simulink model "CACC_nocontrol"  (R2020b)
settings: Solver=FixedStepAuto  StartTime=0.0  StopTime=runtime  FixedStep=stepsize  RelTol=1e-3
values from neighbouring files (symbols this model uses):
  A = [[A_l zeros(3)];[zeros(3) A_f]]    [set_CACC_nocontrol.m]
  A_22s = -eye(4)*0.1    [set_CACC_nocontrol.m]
  A_c = -1/h    (= -1.42857142857)    [set_CACC_nocontrol.m]
  attack_dur = 10    [set_CACC_nocontrol.m]
  attack_mag = 2.8    [set_CACC_nocontrol.m]    (also in Simulation_Main.m = sweep)
  attack_time = 2    [set_CACC_nocontrol.m]
  B = [[B_l zeros(3,1)];[zeros(3,1) B_f]]    [set_CACC_nocontrol.m]
  B_c = [kp/h kd/h -kp -kd]    [set_CACC_nocontrol.m]
  C = [[1 0 0 -1 0 0];[0 1 0 0 -1 0];[0 0 0 0 1 0];[0 0 0 0 0 1]]    [set_CACC_nocontrol.m]
  C_c = 1    [set_CACC_nocontrol.m]
  const = kp/h*r    (= 0.428571428571)    [set_CACC_nocontrol.m]
  D_c = [1/h 0]    [set_CACC_nocontrol.m]
  e2dot_max = diag(M)+U_max    [set_CACC_nocontrol.m]
  e2dot_min = diag(M)-U_max    [set_CACC_nocontrol.m]
  input_mag = 1    [set_CACC_nocontrol.m]
  input_time = [1 6]    [set_CACC_nocontrol.m]
  K = 0.1*eye(4)    [set_CACC_nocontrol.m]    (also in Simulation_Main.m = parameters{1}{2})
  L_f = 4    [set_CACC_nocontrol.m]
  M = diag([2.3500 3.300 2.160 3.6000])    [set_CACC_nocontrol.m]    (also in Simulation_Main.m = parameters{1}{1})
  r = 1.5    [set_CACC_nocontrol.m]
  r_e = e2dot_max./e2dot_min    [set_CACC_nocontrol.m]
  stepsize = 1/1000    (= 0.001)    [set_CACC_nocontrol.m]
  t_max = 2*F*zeta2_max./e2dot_min    [set_CACC_nocontrol.m]
  Thatx_0 = [zeros(2,1);temp(3:end)]    [set_CACC_nocontrol.m]
  U_max = abs(A_22s*obs.F)*abs(zeta2_max)+     abs((obs.A_22-A_22s)*obs.F)*abs(zeta2_max)+     abs(obs.E_2)*abs(zeta1_max)+     abs(obs.A_21*pinv(obs.A_11)*obs.A_12*obs.F)*abs(zeta2_max)+     abs(obs.A_21*pinv(obs.A_11)*obs.E_1)*abs(zeta1_max)    [set_CACC_nocontrol.m]
  x_0 = [-40;15;0;-50;15;0]    [set_CACC_nocontrol.m]
  zeta1_max = abs(tau_l/obs.hattau_l-1)*2*maxacc_l    [set_CACC_nocontrol.m]
  zeta2_max = 3*sqrt(sensor.var)    [set_CACC_nocontrol.m]
undefined symbols (not defined in the file or in its folder): obs, pinv, sensor
libraries: simulink x3

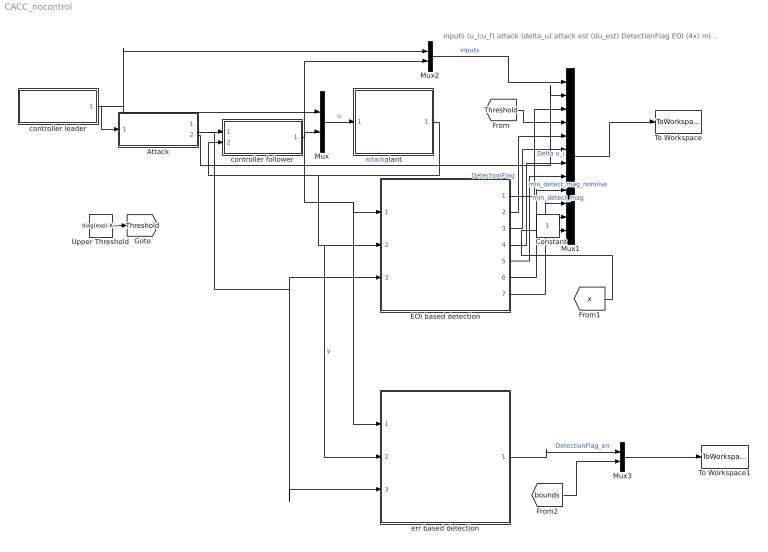
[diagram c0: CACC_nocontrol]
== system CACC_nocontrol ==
  note: inputs (u_l;u_f) attack (delta_u) attack est (du_est) DetectionFlag EOI (4x) min detect mag nonoise min detect mag (old output) x
  Attack : Subsystem
  Constant : Constant
  EOI based detection : Subsystem
  Mux : Mux  Inputs=2
  Mux1 : Mux  Inputs=[2 1 1 4 1 4 1 1 4 4 1 6]
  Mux2 : Mux  Inputs=2
  Mux3 : Mux  Inputs=[1 8]
  To Workspace : ToWorkspace  VariableName=simout  SaveFormat=Structure With Time  SampleTime=-1
  To Workspace1 : ToWorkspace  VariableName=simout_err  SaveFormat=Structure With Time  SampleTime=-1
  Upper Threshold : Constant  Value=diag(exp(-K*t_max))*U_max+(eye(4)-diag(exp(-K*t_max)))*diag(M)
  controller follower : Subsystem
  controller leader : Subsystem
  err based detection : Subsystem
  plant : Subsystem
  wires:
  controller leader/1(u_l) -> Mux2/1, Mux/1, Attack/1(u_l)
  Attack/1(u_l,r) -> err based detection/3(u_l,r), EOI based detection/3(u_l,r), controller follower/1(u_l,r)
  plant/1(y_f) -> err based detection/2(y_f), EOI based detection/2(y_f), controller follower/2(y)  "y"
  controller follower/1(u_f) -> Mux2/2, Mux/2, err based detection/1(u_f), EOI based detection/1(u_f)
  Mux/1 -> plant/1(u)  "u"
  EOI based detection/1(Delta u_l) -> Mux1/3  "Delta u_l"
  EOI based detection/2(Detect_flag) -> Mux1/5  "DetectionFlag"
  Mux2/1 -> Mux1/1  "inputs"
  Mux1/1 -> To Workspace/1
  Attack/2(attack) -> Mux1/2  "attack"
  EOI based detection/3(EOI) -> Mux1/6
  EOI based detection/4(min_detect_mag_nonoise) -> Mux1/7  "min_detect_mag_nonoise"
  EOI based detection/5(min_detect_mag) -> Mux1/8  "min_detect_mag"
  Upper Threshold/1 -> [Threshold]
  [Threshold] -> Mux1/4
  EOI based detection/6(combined+) -> Mux1/9
  EOI based detection/7(combined-) -> Mux1/10
  [x] -> Mux1/12
  err based detection/1(Detect_flag) -> Mux3/1  "DetectionFlag_err"
  [bounds] -> Mux3/2
  Mux3/1 -> To Workspace1/1
  Constant/1 -> Mux1/11

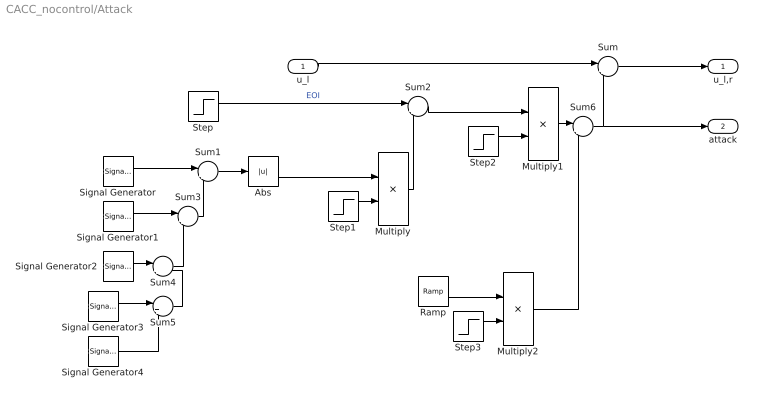
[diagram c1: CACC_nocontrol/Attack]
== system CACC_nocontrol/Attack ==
  u_l : Inport
  Abs : Abs
  Multiply : Product
  Multiply1 : Product
  Multiply2 : Product
  Ramp : simulink/Sources/Ramp  slope=attack_mag/2.4/attack_dur  start=attack_time+3.5*attack_dur  InitialOutput=0
  Signal Generator : SignalGenerator  Amplitude=0.05  Frequency=0.15
  Signal Generator1 : SignalGenerator  Amplitude=0.1  Frequency=0.2
  Signal Generator2 : SignalGenerator  Amplitude=0.05  Frequency=0.05
  Signal Generator3 : SignalGenerator  WaveForm=square  Amplitude=0.1  Frequency=0.005
  Signal Generator4 : SignalGenerator  WaveForm=square  Amplitude=-0.1  Frequency=0.5
  Step : Step  Time=attack_time  After=attack_mag  SampleTime=0
  Step1 : Step  Time=attack_time  After=attack_mag  SampleTime=0
  Step2 : Step  Time=attack_time+attack_dur  Before=1  After=0  SampleTime=0
  Step3 : Step  Time=attack_time+5.5*attack_dur  Before=1  After=0  SampleTime=0
  Sum{,1..6} (7 alike) : Sum  Inputs=|++
  u_l,r : Outport  VectorParamsAs1DForOutWhenUnconnected=off
  attack : Outport  Port=2  VectorParamsAs1DForOutWhenUnconnected=off
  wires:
  u_l/1 -> Sum/1
  Sum/1 -> u_l,r/1
  Sum6/1 -> Sum/2, attack/1
  Signal Generator/1 -> Sum1/1
  Signal Generator1/1 -> Sum3/1
  Sum1/1 -> Abs/1
  Abs/1 -> Multiply/1
  Multiply/1 -> Sum2/2
  Step/1 -> Sum2/1  "EOI"
  Signal Generator2/1 -> Sum4/1
  Sum3/1 -> Sum1/2
  Sum4/1 -> Sum3/2
  Signal Generator3/1 -> Sum5/1
  Sum5/1 -> Sum4/2
  Signal Generator4/1 -> Sum5/2
  Step1/1 -> Multiply/2
  Step2/1 -> Multiply1/2
  Sum2/1 -> Multiply1/1
  Multiply1/1 -> Sum6/1
  Multiply2/1 -> Sum6/2
  Step3/1 -> Multiply2/2
  Ramp/1 -> Multiply2/1

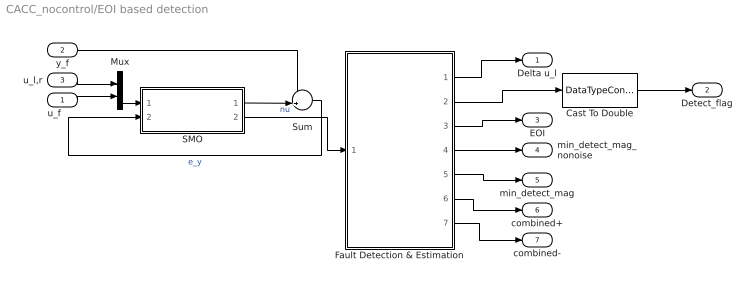
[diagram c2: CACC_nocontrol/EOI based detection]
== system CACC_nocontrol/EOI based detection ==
  u_f : Inport
  y_f : Inport  Port=2
  u_l,r : Inport  Port=3
  Cast To Double : DataTypeConversion  OutDataTypeStr=double
  Fault Detection & Estimation : Subsystem
  Mux : Mux  Inputs=2
  SMO : Subsystem
  Sum : Sum  Inputs=-+|
  Delta u_l : Outport  VectorParamsAs1DForOutWhenUnconnected=off
  Detect_flag : Outport  Port=2  VectorParamsAs1DForOutWhenUnconnected=off
  EOI : Outport  Port=3  VectorParamsAs1DForOutWhenUnconnected=off
  min_detect_mag_nonoise : Outport  Port=4  VectorParamsAs1DForOutWhenUnconnected=off
  min_detect_mag : Outport  Port=5  VectorParamsAs1DForOutWhenUnconnected=off
  combined+ : Outport  Port=6  VectorParamsAs1DForOutWhenUnconnected=off
  combined- : Outport  Port=7  VectorParamsAs1DForOutWhenUnconnected=off
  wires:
  y_f/1 -> Sum/1
  SMO/1(y_hat) -> Sum/2
  Sum/1 -> SMO/2(e_y)  "e_y"
  SMO/2(nu) -> Fault Detection & Estimation/1(nu)  "nu"
  Fault Detection & Estimation/1(Delta u) -> Delta u_l/1
  Fault Detection & Estimation/2(Detection flag) -> Cast To Double/1
  u_l,r/1 -> Mux/1
  Mux/1 -> SMO/1(u)
  u_f/1 -> Mux/2
  Fault Detection & Estimation/3(EOI) -> EOI/1
  Fault Detection & Estimation/5(min_detect_mag) -> min_detect_mag/1
  Fault Detection & Estimation/4(min_detect_mag_nonoise) -> min_detect_mag_nonoise/1
  Cast To Double/1 -> Detect_flag/1
  Fault Detection & Estimation/7(combined-) -> combined-/1
  Fault Detection & Estimation/6(combined+) -> combined+/1

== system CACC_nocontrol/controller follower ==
  u_l,r : Inport
  y : Inport  Port=2
  Constant : Constant  Value=const
  Gain : Gain  Gain=A_c  Multiplication=Matrix(K*u)
  Gain1 : Gain  Gain=B_c  Multiplication=Matrix(K*u)
  Gain2 : Gain  Gain=C_c  Multiplication=Matrix(K*u)
  Gain3 : Gain  Gain=D_c(1)  Multiplication=Matrix(K*u)
  Integrator : Integrator
  Sum : Sum  Inputs=++++
  u_f : Outport  VectorParamsAs1DForOutWhenUnconnected=off
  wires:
  y/1 -> Gain1/1
  Gain1/1 -> Sum/3
  Integrator/1 -> Gain2/1, Gain/1
  Gain/1 -> Sum/4
  Sum/1 -> Integrator/1
  Gain2/1 -> u_f/1
  Constant/1 -> Sum/1
  u_l,r/1 -> Gain3/1
  Gain3/1 -> Sum/2

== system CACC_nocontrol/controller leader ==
  Step : Step  Time=input_time(1)  After=input_mag  SampleTime=0
  Step1 : Step  Time=input_time(2)  After=-input_mag  SampleTime=0
  Step2 : Step  Time=35  After=-input_mag  SampleTime=0
  Step3 : Step  Time=40  After=input_mag  SampleTime=0
  Sum : Sum  Inputs=|++
  Sum2 : Sum  Inputs=|++
  Sum3 : Sum  Inputs=++|
  u_l : Outport  VectorParamsAs1DForOutWhenUnconnected=off
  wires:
  Step/1 -> Sum/1
  Sum3/1 -> u_l/1
  Step1/1 -> Sum/2
  Step3/1 -> Sum2/2
  Step2/1 -> Sum2/1
  Sum/1 -> Sum3/2
  Sum2/1 -> Sum3/1

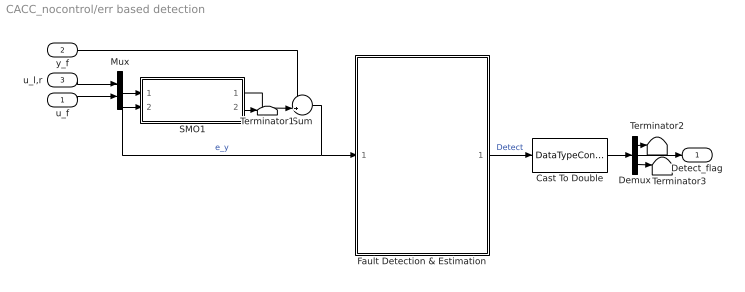
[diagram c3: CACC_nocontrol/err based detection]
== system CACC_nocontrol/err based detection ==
  u_f : Inport
  y_f : Inport  Port=2
  u_l,r : Inport  Port=3
  Cast To Double : DataTypeConversion  OutDataTypeStr=double
  Demux : Demux  Outputs=[1 1 2]
  Fault Detection & Estimation : Subsystem
  Mux : Mux  Inputs=2
  SMO1 : Subsystem
  Sum : Sum  Inputs=-+|
  Terminator1 : Terminator
  Terminator2 : Terminator
  Terminator3 : Terminator
  Detect_flag : Outport  VectorParamsAs1DForOutWhenUnconnected=off
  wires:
  y_f/1 -> Sum/1
  Sum/1 -> SMO1/2(e_y), Fault Detection & Estimation/1(e_y)  "e_y"
  u_l,r/1 -> Mux/1
  u_f/1 -> Mux/2
  Fault Detection & Estimation/1(Detection) -> Cast To Double/1  "Detect"
  Cast To Double/1 -> Demux/1
  Demux/2 -> Detect_flag/1
  Mux/1 -> SMO1/1(u)
  SMO1/1(y_hat) -> Sum/2
  SMO1/2(nu) -> Terminator1/1
  Demux/1 -> Terminator2/1
  Demux/3 -> Terminator3/1

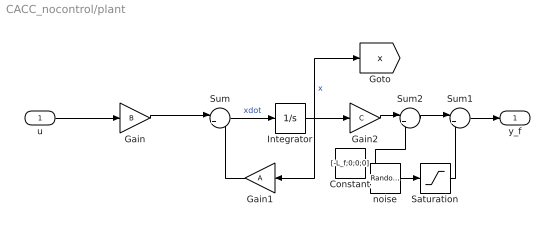
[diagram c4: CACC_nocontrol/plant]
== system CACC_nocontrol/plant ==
  u : Inport
  Constant : Constant  Value=[-L_f;0;0;0]
  Gain : Gain  Gain=B  Multiplication=Matrix(K*u)
  Gain1 : Gain  Gain=A  Multiplication=Matrix(K*u)
  Gain2 : Gain  Gain=C  Multiplication=Matrix(K*u)
  Integrator : Integrator  InitialCondition=x_0
  Saturation : Saturate  UpperLimit=zeta2_max  LowerLimit=-zeta2_max
  Sum : Sum  Inputs=|++
  Sum1 : Sum  Inputs=|++
  Sum2 : Sum  Inputs=|++
  noise : RandomNumber  Mean=zeros(4,1)  Variance=sensor.var  Seed=[5;1423;145;23]  SampleTime=0
  y_f : Outport  VectorParamsAs1DForOutWhenUnconnected=off
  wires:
  u/1 -> Gain/1
  Integrator/1 -> [x], Gain2/1, Gain1/1  "x"
  Gain/1 -> Sum/1
  Gain1/1 -> Sum/2
  Sum/1 -> Integrator/1  "xdot"
  Gain2/1 -> Sum2/1
  Sum1/1 -> y_f/1
  noise/1 -> Saturation/1
  Sum2/1 -> Sum1/1
  Constant/1 -> Sum2/2
  Saturation/1 -> Sum1/2

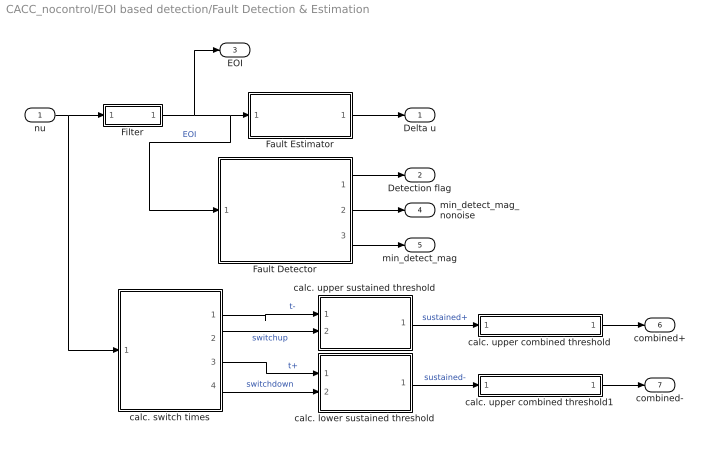
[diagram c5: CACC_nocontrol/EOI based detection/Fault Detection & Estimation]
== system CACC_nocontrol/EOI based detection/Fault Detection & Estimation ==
  nu : Inport
  Fault Detector : Subsystem
  Fault Estimator : Subsystem
  Filter : Subsystem
  calc. lower sustained threshold : Subsystem
  calc. switch times : Subsystem
  calc. upper combined threshold : Subsystem
  calc. upper combined threshold1 : Subsystem
  calc. upper sustained threshold : Subsystem
  Delta u : Outport  VectorParamsAs1DForOutWhenUnconnected=off
  Detection flag : Outport  Port=2  VectorParamsAs1DForOutWhenUnconnected=off
  EOI : Outport  Port=3  VectorParamsAs1DForOutWhenUnconnected=off
  min_detect_mag_nonoise : Outport  Port=4  VectorParamsAs1DForOutWhenUnconnected=off
  min_detect_mag : Outport  Port=5  VectorParamsAs1DForOutWhenUnconnected=off
  combined+ : Outport  Port=6  VectorParamsAs1DForOutWhenUnconnected=off
  combined- : Outport  Port=7  VectorParamsAs1DForOutWhenUnconnected=off
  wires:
  Fault Estimator/1(Delta u) -> Delta u/1
  nu/1 -> calc. switch times/1(nu), Filter/1(nu)
  Fault Detector/1(flag) -> Detection flag/1
  Filter/1(EOI) -> EOI/1, Fault Detector/1(EOI), Fault Estimator/1(EOI)  "EOI"
  Fault Detector/2(min_detect_fault_nonoise) -> min_detect_mag_nonoise/1
  Fault Detector/3(min_detect_fault) -> min_detect_mag/1
  calc. switch times/3(t+) -> calc. lower sustained threshold/1(t+)  "t+"
  calc. switch times/4(switchdown) -> calc. lower sustained threshold/2(switchdown)  "switchdown"
  calc. switch times/1(t-) -> calc. upper sustained threshold/1(t-)  "t-"
  calc. switch times/2(switchup) -> calc. upper sustained threshold/2(switchup)  "switchup"
  calc. upper sustained threshold/1(Sustained+) -> calc. upper combined threshold/1(Sustained+)  "sustained+"
  calc. lower sustained threshold/1(Sustained-) -> calc. upper combined threshold1/1(Sustained-)  "sustained-"
  calc. upper combined threshold/1(Combined+) -> combined+/1
  calc. upper combined threshold1/1(Combined-) -> combined-/1

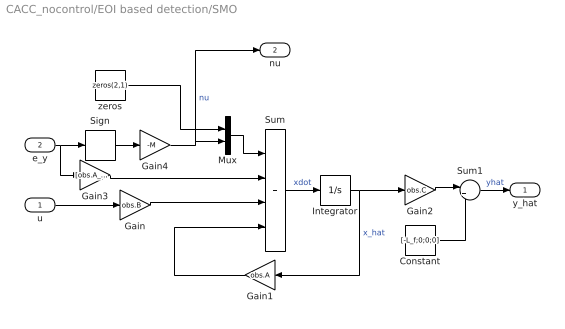
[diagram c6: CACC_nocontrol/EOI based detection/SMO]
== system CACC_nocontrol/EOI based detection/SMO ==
  u : Inport
  e_y : Inport  Port=2
  Constant : Constant  Value=[-L_f;0;0;0]
  Gain : Gain  Gain=obs.B  Multiplication=Matrix(K*u)
  Gain1 : Gain  Gain=obs.A  Multiplication=Matrix(K*u)
  Gain2 : Gain  Gain=obs.C  Multiplication=Matrix(K*u)
  Gain3 : Gain  Gain=[obs.A_12;obs.A_22-A_22s]  Multiplication=Matrix(K*u)
  Gain4 : Gain  Gain=-M  Multiplication=Matrix(K*u)
  Integrator : Integrator  InitialCondition=Thatx_0%[r;0;0;0;0;0]
  Mux : Mux  Inputs=[2 4]
  Sign : Signum
  Sum : Sum  Inputs=++++
  Sum1 : Sum  Inputs=|++
  zeros : Constant  Value=zeros(2,1)
  y_hat : Outport  VectorParamsAs1DForOutWhenUnconnected=off
  nu : Outport  Port=2  VectorParamsAs1DForOutWhenUnconnected=off
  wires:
  u/1 -> Gain/1
  Sum/1 -> Integrator/1  "xdot"
  Integrator/1 -> Gain2/1, Gain1/1  "x_hat"
  Gain/1 -> Sum/3
  Gain1/1 -> Sum/4
  Gain2/1 -> Sum1/1
  Gain3/1 -> Sum/2
  e_y/1 -> Gain3/1, Sign/1
  Sign/1 -> Gain4/1
  Gain4/1 -> Mux/2, nu/1  "nu"
  zeros/1 -> Mux/1
  Mux/1 -> Sum/1
  Sum1/1 -> y_hat/1  "yhat"
  Constant/1 -> Sum1/2

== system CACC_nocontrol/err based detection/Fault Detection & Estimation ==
  e_y : Inport
  Less Than1 : RelationalOperator  Operator=<  OutDataTypeStr=boolean  RndMeth=Simplest
  Mux : Mux  Inputs=[4 4]
  calc. lower bound : Subsystem
  calc. upper bound : Subsystem
  Detection : Outport  VectorParamsAs1DForOutWhenUnconnected=off
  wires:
  e_y/1 -> calc. lower bound/1(e_y), calc. upper bound/1(e_y)  "e_y"
  Less Than1/1 -> Detection/1
  calc. upper bound/1(bound) -> Less Than1/1, Mux/1  "bound+"
  calc. lower bound/1(bound) -> Less Than1/2, Mux/2  "bound-"
  Mux/1 -> [bounds]

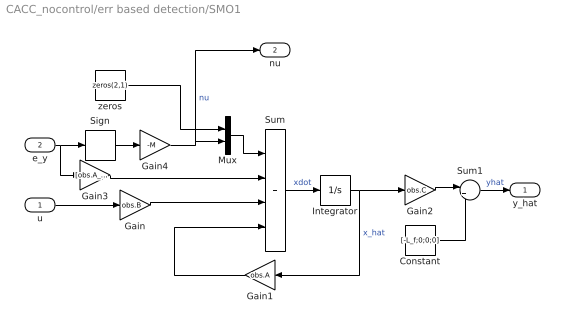
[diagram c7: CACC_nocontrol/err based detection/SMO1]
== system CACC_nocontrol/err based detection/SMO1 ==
  u : Inport
  e_y : Inport  Port=2
  Constant : Constant  Value=[-L_f;0;0;0]
  Gain : Gain  Gain=obs.B  Multiplication=Matrix(K*u)
  Gain1 : Gain  Gain=obs.A  Multiplication=Matrix(K*u)
  Gain2 : Gain  Gain=obs.C  Multiplication=Matrix(K*u)
  Gain3 : Gain  Gain=[obs.A_12;obs.A_22-A_22s]  Multiplication=Matrix(K*u)
  Gain4 : Gain  Gain=-M  Multiplication=Matrix(K*u)
  Integrator : Integrator  InitialCondition=Thatx_0%[r;0;0;0;0;0]
  Mux : Mux  Inputs=[2 4]
  Sign : Signum
  Sum : Sum  Inputs=++++
  Sum1 : Sum  Inputs=|++
  zeros : Constant  Value=zeros(2,1)
  y_hat : Outport  VectorParamsAs1DForOutWhenUnconnected=off
  nu : Outport  Port=2  VectorParamsAs1DForOutWhenUnconnected=off
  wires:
  u/1 -> Gain/1
  Sum/1 -> Integrator/1  "xdot"
  Integrator/1 -> Gain2/1, Gain1/1  "x_hat"
  Gain/1 -> Sum/3
  Gain1/1 -> Sum/4
  Gain2/1 -> Sum1/1
  Gain3/1 -> Sum/2
  e_y/1 -> Gain3/1, Sign/1
  Sign/1 -> Gain4/1
  Gain4/1 -> Mux/2, nu/1  "nu"
  zeros/1 -> Mux/1
  Mux/1 -> Sum/1
  Sum1/1 -> y_hat/1  "yhat"
  Constant/1 -> Sum1/2

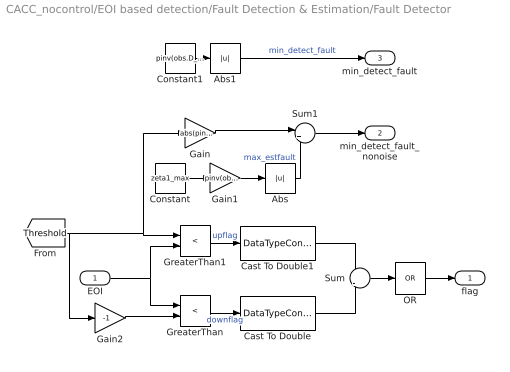
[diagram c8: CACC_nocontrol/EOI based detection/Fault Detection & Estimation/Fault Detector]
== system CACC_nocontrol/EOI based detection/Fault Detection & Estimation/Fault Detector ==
  EOI : Inport
  Abs : Abs
  Abs1 : Abs
  Cast To Double : DataTypeConversion  OutDataTypeStr=double
  Cast To Double1 : DataTypeConversion  OutDataTypeStr=double
  Constant : Constant  Value=zeta1_max
  Constant1 : Constant  Value=pinv(obs.D_2-obs.A_21*pinv(obs.A_11)*obs.D_1)*((eye(4)+diag(exp(-K*t_max)))*U_max+(eye(4)-diag(exp(-K*t_max)))*diag(M))
  Gain : Gain  Gain=abs(pinv(obs.D_2-obs.A_21*pinv(obs.A_11)*obs.D_1))  Multiplication=Matrix(K*u)
  Gain1 : Gain  Gain=pinv(obs.D_2-obs.A_21*pinv(obs.A_11)*obs.D_1)*-(obs.A_21*pinv(obs.A_11)*abs(obs.E_1)+abs(obs.E_2))  Multiplication=Matrix(K*u)
  Gain2 : Gain  Gain=-1
  GreaterThan : RelationalOperator  Operator=<  RndMeth=Simplest
  GreaterThan1 : RelationalOperator  Operator=<  OutDataTypeStr=boolean  RndMeth=Simplest
  OR : Logic  Operator=OR  Inputs=1  IconShape=distinctive  AllPortsSameDT=off  OutDataTypeStr=boolean
  Sum : Sum  Inputs=+|-
  Sum1 : Sum  Inputs=|++
  flag : Outport  VectorParamsAs1DForOutWhenUnconnected=off
  min_detect_fault_nonoise : Outport  Port=2  VectorParamsAs1DForOutWhenUnconnected=off
  min_detect_fault : Outport  Port=3  VectorParamsAs1DForOutWhenUnconnected=off
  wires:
  Sum/1 -> OR/1
  [Threshold] -> Gain2/1, Gain/1, GreaterThan1/1
  Gain2/1 -> GreaterThan/2
  EOI/1 -> GreaterThan1/2, GreaterThan/1
  GreaterThan/1 -> Cast To Double/1  "downflag"
  GreaterThan1/1 -> Cast To Double1/1  "upflag"
  Cast To Double/1 -> Sum/2
  Cast To Double1/1 -> Sum/1
  Gain/1 -> Sum1/1
  Constant/1 -> Gain1/1
  Gain1/1 -> Abs/1
  Sum1/1 -> min_detect_fault_nonoise/1
  Abs/1 -> Sum1/2  "max_estfault"
  Constant1/1 -> Abs1/1
  Abs1/1 -> min_detect_fault/1  "min_detect_fault"
  OR/1 -> flag/1

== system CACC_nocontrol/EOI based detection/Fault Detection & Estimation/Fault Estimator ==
  EOI : Inport
  Gain : Gain  Gain=pinv(-obs.A_21*pinv(obs.A_11)*obs.D_1+obs.D_2)  Multiplication=Matrix(K*u)
  Delta u : Outport  VectorParamsAs1DForOutWhenUnconnected=off
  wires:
  EOI/1 -> Gain/1
  Gain/1 -> Delta u/1

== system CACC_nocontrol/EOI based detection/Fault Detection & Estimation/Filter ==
  nu : Inport
  Gain : Gain  Gain=K  Multiplication=Matrix(K*u)
  Integrator : Integrator
  Sum : Sum  Inputs=|+-
  EOI : Outport  VectorParamsAs1DForOutWhenUnconnected=off
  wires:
  nu/1 -> Sum/1
  Integrator/1 -> Sum/2, EOI/1
  Sum/1 -> Gain/1
  Gain/1 -> Integrator/1

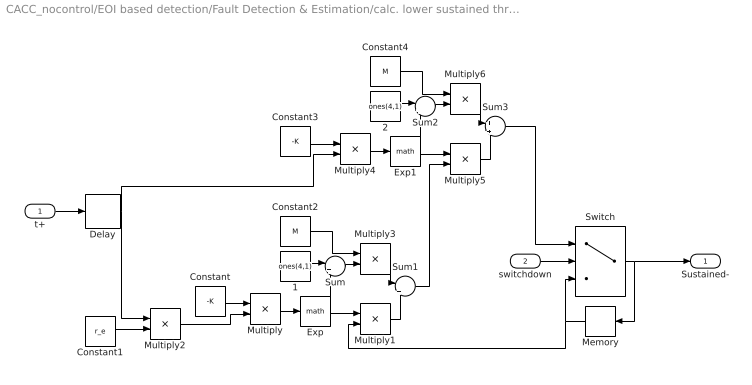
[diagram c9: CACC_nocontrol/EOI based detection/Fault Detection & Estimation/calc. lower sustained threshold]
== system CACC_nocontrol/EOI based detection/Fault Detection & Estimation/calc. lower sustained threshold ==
  t+ : Inport
  switchdown : Inport  Port=2
  1 : Constant  Value=ones(4,1)
  2 : Constant  Value=ones(4,1)
  Constant : Constant  Value=-K
  Constant1 : Constant  Value=r_e
  Constant2 : Constant  Value=M
  Constant3 : Constant  Value=-K
  Constant4 : Constant  Value=M
  Delay : Delay  DelayLength=1
  Exp : Math  SignedPower=on
  Exp1 : Math  SignedPower=on
  Memory : Memory
  Multiply{,3..4,6} (4 alike) : Product  Multiplication=Matrix(*)
  Multiply1 : Product
  Multiply2 : Product
  Multiply5 : Product
  Sum : Sum  Inputs=|+-
  Sum1 : Sum  Inputs=-|+
  Sum2 : Sum  Inputs=|+-
  Sum3 : Sum  Inputs=+|+
  Switch : Switch  Criteria=u2 > Threshold
  Sustained- : Outport  VectorParamsAs1DForOutWhenUnconnected=off
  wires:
  Delay/1 -> Multiply4/2, Multiply2/1
  t+/1 -> Delay/1
  switchdown/1 -> Switch/2
  Switch/1 -> Sustained-/1, Memory/1
  Memory/1 -> Switch/3, Multiply1/2
  Constant/1 -> Multiply/1
  Multiply/1 -> Exp/1
  Exp/1 -> Sum/2, Multiply1/1
  Constant1/1 -> Multiply2/2
  Multiply1/1 -> Sum1/2
  1/1 -> Sum/1
  Sum/1 -> Multiply3/2
  Constant2/1 -> Multiply3/1
  Multiply3/1 -> Sum1/1
  2/1 -> Sum2/1
  Sum1/1 -> Multiply5/2
  Multiply6/1 -> Sum3/1
  Sum2/1 -> Multiply6/2
  Constant4/1 -> Multiply6/1
  Multiply4/1 -> Exp1/1
  Exp1/1 -> Sum2/2, Multiply5/1
  Constant3/1 -> Multiply4/1
  Multiply5/1 -> Sum3/2
  Sum3/1 -> Switch/1
  Multiply2/1 -> Multiply/2

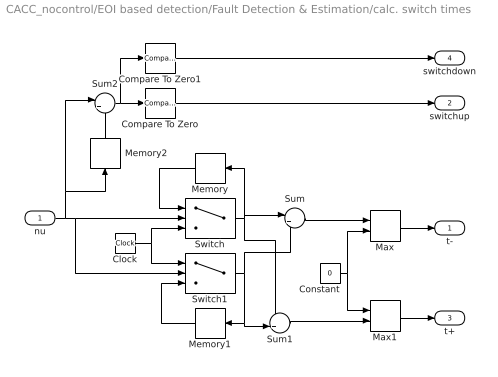
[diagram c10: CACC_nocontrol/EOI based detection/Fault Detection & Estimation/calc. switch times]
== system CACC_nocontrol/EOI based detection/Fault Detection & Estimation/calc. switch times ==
  nu : Inport
  Clock : Clock
  Compare To Zero : simulink/Logic and Bit Operations/Compare To Zero  relop=>  OutDataTypeStr=boolean
  Compare To Zero1 : simulink/Logic and Bit Operations/Compare To Zero  relop=<  OutDataTypeStr=boolean
  Constant : Constant  Value=0
  Max : MinMax  Function=max  Inputs=2
  Max1 : MinMax  Function=max  Inputs=2
  Memory : Memory
  Memory1 : Memory
  Memory2 : Memory
  Sum : Sum  Inputs=|+-
  Sum1 : Sum  Inputs=-+|
  Sum2 : Sum  Inputs=|+-
  Switch : Switch  Criteria=u2 > Threshold
  Switch1 : Switch  Criteria=u2 > Threshold
  t- : Outport  VectorParamsAs1DForOutWhenUnconnected=off
  switchup : Outport  Port=2  VectorParamsAs1DForOutWhenUnconnected=off
  t+ : Outport  Port=3  VectorParamsAs1DForOutWhenUnconnected=off
  switchdown : Outport  Port=4  VectorParamsAs1DForOutWhenUnconnected=off
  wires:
  Clock/1 -> Switch1/1, Switch/3
  Switch/1 -> Sum/1, Sum1/1, Memory/1
  Memory/1 -> Switch/1
  Switch1/1 -> Sum1/2, Memory1/1, Sum/2
  Memory1/1 -> Switch1/3
  Sum/1 -> Max/1
  Constant/1 -> Max/2, Max1/1
  Max/1 -> t-/1
  Sum1/1 -> Max1/2
  Max1/1 -> t+/1
  Memory2/1 -> Sum2/2
  nu/1 -> Memory2/1, Sum2/1, Switch/2, Switch1/2
  Sum2/1 -> Compare To Zero1/1, Compare To Zero/1
  Compare To Zero/1 -> switchup/1
  Compare To Zero1/1 -> switchdown/1

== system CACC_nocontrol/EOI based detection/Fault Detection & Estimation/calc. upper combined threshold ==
  Sustained+ : Inport
  1 : Constant  Value=ones(4,1)
  Constant1 : Constant  Value=exp(-K*t_max)
  Constant2 : Constant  Value=M
  Multiply1 : Product
  Multiply3 : Product  Multiplication=Matrix(*)
  Sum : Sum  Inputs=|+-
  Sum1 : Sum  Inputs=+|+
  Combined+ : Outport  VectorParamsAs1DForOutWhenUnconnected=off
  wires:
  Multiply3/1 -> Sum1/1
  Sum/1 -> Multiply3/2
  Constant2/1 -> Multiply3/1
  1/1 -> Sum/1
  Sustained+/1 -> Multiply1/2
  Constant1/1 -> Sum/2, Multiply1/1
  Multiply1/1 -> Sum1/2
  Sum1/1 -> Combined+/1

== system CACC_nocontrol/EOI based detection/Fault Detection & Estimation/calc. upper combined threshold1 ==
  Sustained- : Inport
  1 : Constant  Value=ones(4,1)
  Constant1 : Constant  Value=exp(-K*t_max)
  Constant2 : Constant  Value=M
  Multiply1 : Product
  Multiply3 : Product  Multiplication=Matrix(*)
  Sum : Sum  Inputs=|+-
  Sum1 : Sum  Inputs=-|+
  Combined- : Outport  VectorParamsAs1DForOutWhenUnconnected=off
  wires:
  Multiply3/1 -> Sum1/1
  Sum/1 -> Multiply3/2
  Constant2/1 -> Multiply3/1
  1/1 -> Sum/1
  Sustained-/1 -> Multiply1/2
  Constant1/1 -> Sum/2, Multiply1/1
  Multiply1/1 -> Sum1/2
  Sum1/1 -> Combined-/1

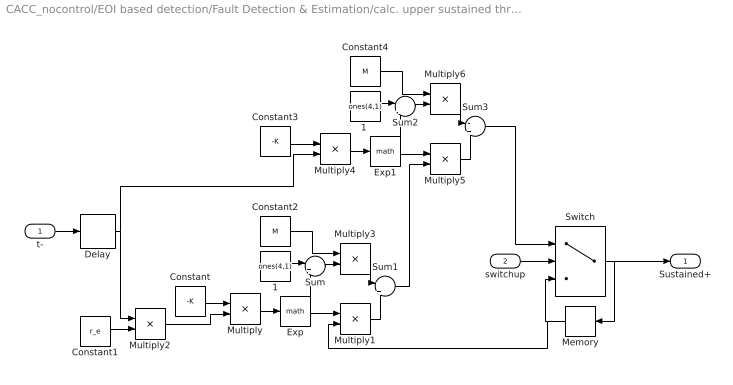
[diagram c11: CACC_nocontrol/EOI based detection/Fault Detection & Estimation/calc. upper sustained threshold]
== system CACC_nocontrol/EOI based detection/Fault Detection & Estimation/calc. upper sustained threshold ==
  t- : Inport
  switchup : Inport  Port=2
  1 : Constant  Value=ones(4,1)
  "1 " : Constant  Value=ones(4,1)
  Constant : Constant  Value=-K
  Constant1 : Constant  Value=r_e
  Constant2 : Constant  Value=M
  Constant3 : Constant  Value=-K
  Constant4 : Constant  Value=M
  Delay : Delay  DelayLength=1
  Exp : Math  SignedPower=on
  Exp1 : Math  SignedPower=on
  Memory : Memory
  Multiply{,3..4,6} (4 alike) : Product  Multiplication=Matrix(*)
  Multiply1 : Product
  Multiply2 : Product
  Multiply5 : Product
  Sum : Sum  Inputs=|+-
  Sum1 : Sum  Inputs=+|+
  Sum2 : Sum  Inputs=|+-
  Sum3 : Sum  Inputs=-|+
  Switch : Switch  Criteria=u2 > Threshold
  Sustained+ : Outport  VectorParamsAs1DForOutWhenUnconnected=off
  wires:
  Delay/1 -> Multiply4/2, Multiply2/1
  t-/1 -> Delay/1
  switchup/1 -> Switch/2
  Switch/1 -> Sustained+/1, Memory/1
  Memory/1 -> Multiply1/2, Switch/3
  Sum3/1 -> Switch/1
  Constant/1 -> Multiply/1
  Multiply/1 -> Exp/1
  Exp/1 -> Sum/2, Multiply1/1
  Constant1/1 -> Multiply2/2
  Multiply1/1 -> Sum1/2
  1/1 -> Sum/1
  Sum/1 -> Multiply3/2
  Constant2/1 -> Multiply3/1
  Multiply3/1 -> Sum1/1
  "1 "/1 -> Sum2/1
  Sum1/1 -> Multiply5/2
  Multiply6/1 -> Sum3/1
  Sum2/1 -> Multiply6/2
  Constant4/1 -> Multiply6/1
  Multiply4/1 -> Exp1/1
  Exp1/1 -> Sum2/2, Multiply5/1
  Constant3/1 -> Multiply4/1
  Multiply5/1 -> Sum3/2
  Multiply2/1 -> Multiply/2

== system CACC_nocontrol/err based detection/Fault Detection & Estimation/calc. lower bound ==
  e_y : Inport
  Delay2 : Delay  DelayLength=1  InitialConditionSource=Input port  InitialCondition=-abs(obs.F)*abs(zeta2_max)
  Min : MinMax  Function=max  Inputs=3
  Min1 : MinMax  Function=max  Inputs=2
  Sum : Sum  Inputs=|++
  Sum1 : Sum  Inputs=++|
  min_noise : Constant  Value=-abs(obs.F)*abs(zeta2_max)
  minmax_diff : Subsystem
  bound : Outport  VectorParamsAs1DForOutWhenUnconnected=off
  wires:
  Min/1 -> Sum1/1, bound/1
  minmax_diff/1(diff) -> Sum1/2
  Sum1/1 -> Delay2/1
  Delay2/1 -> Min/1  "diff_bound-"
  e_y/1 -> minmax_diff/1(e_y), Sum/1
  Sum/1 -> Min1/2, Min/2  "noisebound-"
  min_noise/1 -> Min/3, Min1/1, Sum/2  "min noise"
  Min1/1 -> Delay2/2

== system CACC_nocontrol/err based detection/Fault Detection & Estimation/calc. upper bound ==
  e_y : Inport
  Delay2 : Delay  DelayLength=1  InitialConditionSource=Input port  InitialCondition=abs(obs.F)*abs(zeta2_max)
  Min : MinMax  Inputs=3
  Min1 : MinMax  Inputs=2
  Sum : Sum  Inputs=|++
  Sum1 : Sum  Inputs=++|
  max_noise : Constant  Value=abs(obs.F)*abs(zeta2_max)
  minmax_diff : Subsystem
  bound : Outport  VectorParamsAs1DForOutWhenUnconnected=off
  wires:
  minmax_diff/1(diff) -> Sum1/2
  Sum1/1 -> Delay2/1
  Delay2/1 -> Min/1  "diff_bound"
  e_y/1 -> Sum/1, minmax_diff/1(e_y)
  Sum/1 -> Min1/1, Min/2  "noisebound"
  max_noise/1 -> Sum/2, Min1/2, Min/3  "max noise"
  Min1/1 -> Delay2/2
  Min/1 -> Sum1/1, bound/1

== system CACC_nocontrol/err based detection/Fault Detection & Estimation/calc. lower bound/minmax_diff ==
  e_y : Inport
  Constant : Constant  Value=e2dot_min
  Constant3 : Constant  Value=-e2dot_max
  Gain : Gain  Gain=stepsize
  Switch : Switch  Criteria=u2 > Threshold  Threshold=[0;0;0;0]
  diff : Outport  VectorParamsAs1DForOutWhenUnconnected=off
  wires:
  Constant/1 -> Switch/3
  Switch/1 -> Gain/1  "switchresp"
  e_y/1 -> Switch/2
  Constant3/1 -> Switch/1
  Gain/1 -> diff/1  "switchrespgain"

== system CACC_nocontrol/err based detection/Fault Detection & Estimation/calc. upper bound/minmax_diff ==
  e_y : Inport
  Constant : Constant  Value=e2dot_max
  Constant3 : Constant  Value=-e2dot_min
  Gain : Gain  Gain=stepsize
  Switch : Switch  Criteria=u2 > Threshold  Threshold=[0;0;0;0]
  diff : Outport  VectorParamsAs1DForOutWhenUnconnected=off
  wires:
  Constant/1 -> Switch/3
  Switch/1 -> Gain/1
  e_y/1 -> Switch/2
  Constant3/1 -> Switch/1
  Gain/1 -> diff/1
